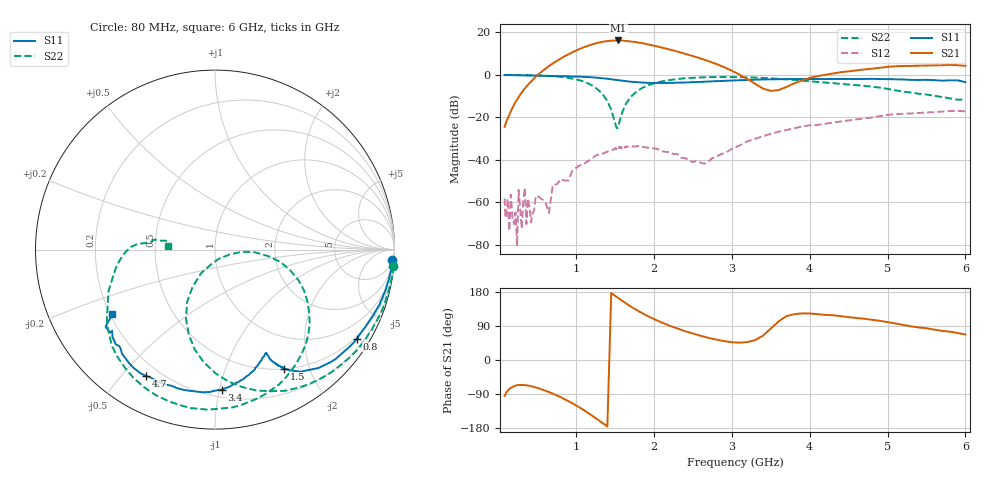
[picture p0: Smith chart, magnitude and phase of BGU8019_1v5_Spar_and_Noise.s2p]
! BGU8019,  Vcc= 1.50 V, Icc= 4.2860 mA
# MHz S MA R 50
!  Freq-MHz  S11-mag  S11-arg  S21-mag  S21-arg  S12-mag  S12-arg  S22-mag  S22-arg
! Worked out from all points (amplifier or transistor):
!   130 points, 80 MHz to 6 GHz, reference 50 ohm
!   highest |S21| = 16.2 dB at 1.54 GHz (marker M1)
!   |S21| within 3 dB of that: 1.112 GHz to 2.063 GHz (951.3 MHz wide, 59.9 % of centre)
!   unconditionally stable (mu >= 1): 136.6 MHz to 248.2 MHz; 271.6 MHz to 314.6 MHz; 350.1 MHz to end of sweep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
!   at 480 MHz: K = 1.59, MAG = 23.6 dB, |S12| = -57.2 dB
!   at 1.615 GHz: K = 1.84, MAG = 19.9 dB, |S12| = -34.3 dB
!   at 6 GHz: K = 1.39, MAG = 7.0 dB, |S12| = -17.2 dB
!   lowest NFmin = 0.39 dB at 1.1 GHz
!   S11 on the Smith chart (normalised r, x): 80 MHz: 7, -34; 800 MHz: 0.44, -3.43; 1.5 GHz: 0.50, -1.63; 3.4 GHz: 0.25, -1.02; 4.7 GHz: 0.15, -0.58; 6 GHz: 0.21, -0.28
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80  0.9888 -3.3  0.05947 -94.8  0.001242 75.0  0.9972 -5.2
140  0.9891 -5.9  0.1164 -76.8  0.0002142 112.7  0.9966 -9.3
160  0.9874 -6.7  0.1401 -73.5  0.001526 -171.7  0.9952 -10.7
240  0.9821 -10.0  0.2621 -66.6  9.364e-05 -96.0  0.9921 -16.1
260  0.9792 -10.9  0.3002 -66.0  0.001966 103.0  0.991 -17.6
300  0.9772 -12.7  0.3838 -65.9  0.0002417 121.1  0.9901 -20.2
340  0.9748 -14.2  0.4783 -66.3  0.002205 103.7  0.9851 -23.1
360  0.9719 -15.0  0.531 -66.8  0.0003106 -23.5  0.9838 -24.5
800  0.9344 -32.0  2.414 -98.1  0.003515 -147.1  0.8985 -59.0
1100  0.8987 -44.2  4.478 -132.5  0.008054 -176.4  0.6901 -89.7
1300  0.8436 -53.0  5.789 -160.7  0.0135 163.6  0.4157 -112.9
1500  0.7677 -59.7  6.432 169.3  0.01877 130.8  0.07343 -98.1
1540  0.7515 -60.6  6.44 163.3  0.01856 127.2  0.06202 -40.0
1800  0.6656 -63.3  5.755 129.0  0.02127 91.9  0.4338 -15.3
2100  0.6431 -63.9  4.385 98.9  0.01594 58.1  0.7018 -42.1
2500  0.6718 -67.9  2.764 69.7  0.008819 -3.9  0.8536 -71.2
3100  0.7472 -79.7  1.009 45.9  0.02189 -128.1  0.8839 -106.8
3400  0.7807 -87.2  0.4755 64.3  0.03629 -153.8  0.8468 -122.4
4100  0.8004 -105.2  0.9321 120.8  0.06622 165.7  0.6775 -152.0
4700  0.8029 -118.7  1.342 108.9  0.09454 147.1  0.5505 -171.4
5100  0.7871 -128.8  1.591 96.4  0.1197 131.5  0.4323 175.9
6000  0.6739 -147.9  1.625 67.3  0.1381 105.5  0.2609 175.3
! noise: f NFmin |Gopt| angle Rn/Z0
1000  0.4043  0.6426  32.27  0.1977
1250  0.4257  0.6075  35.78  0.1923
1505  0.4929  0.5914  43.72  0.1975
1535  0.5283  0.5955  44.7  0.1901
1560  0.5141  0.5938  45.36  0.1885
1590  0.497  0.5814  47.39  0.1878
1620  0.5056  0.5726  48.04  0.195
1645  0.5652  0.5764  47.87  0.182
1900  0.6201  0.5657  52.61  0.2041
2200  0.6597  0.4732  61.48  0.2
